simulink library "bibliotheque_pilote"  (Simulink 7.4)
settings: Solver=ode45  StartTime=0.0  StopTime=10.0  RelTol=1e-3
libraries: fl_lib x20, nesl_utility x7, elec_lib x1

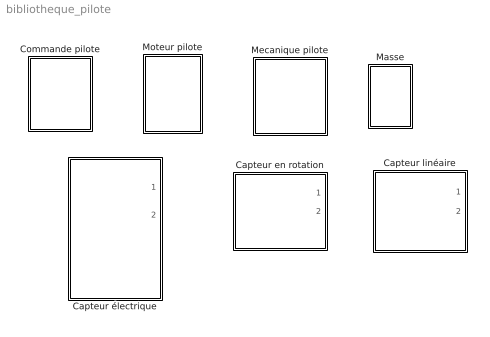
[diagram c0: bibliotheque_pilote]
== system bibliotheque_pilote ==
  Capteur en rotation : Subsystem
  Capteur linéaire : Subsystem
  Capteur électrique : Subsystem
  Commande pilote : Subsystem
  Masse : Subsystem  mask(Masse soulevée par la tige){masse=14}
      mask prompts: masse "Masse en kg"
  Mecanique pilote : Subsystem
  Moteur pilote : Subsystem

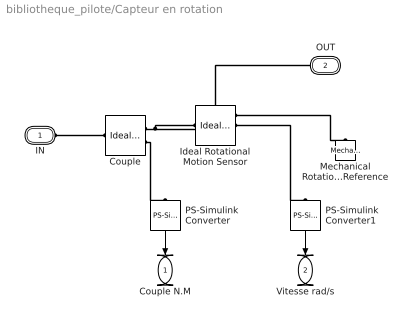
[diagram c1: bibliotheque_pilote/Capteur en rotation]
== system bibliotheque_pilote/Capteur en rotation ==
  Couple : fl_lib/Mechanical/Mechanical Sensors/Ideal Torque Sensor  DialogController=NetworkEngine.DynNeDlgSource  SystemSampleTime=-1  w_Log=off  t_Log=off  LocalVarNames=|w|t  LocalVarDescs=|w|t  LocalVarLogging=[0 0]
  Ideal Rotational Motion Sensor : fl_lib/Mechanical/Mechanical Sensors/Ideal Rotational Motion Sensor  DialogController=NetworkEngine.DynNeDlgSource  SystemSampleTime=-1  offset=0 rad  w_Log=off  t_Log=off  phi_Log=off  LocalVarNames=|w|t|phi  LocalVarDescs=|w|t|phi  LocalVarLogging=[0 0 0]
  Mechanical Rotational Reference : fl_lib/Mechanical/Rotational Elements/Mechanical Rotational Reference  DialogController=NetworkEngine.DynNeDlgSource  SystemSampleTime=-1  t_Log=off  LocalVarNames=|t  LocalVarDescs=|t  LocalVarLogging=0
  PS-Simulink Converter : nesl_utility/PS-Simulink Converter  DialogController=NetworkEngine.DynNeUtilDlgSource  SystemSampleTime=-1  PhysicalDomain=network_engine_domain  LeftPortType=input  RightPortType=output  SubClassName=ps_output  Unit=N*m  AffineConversion=off
  PS-Simulink Converter1 : nesl_utility/PS-Simulink Converter  DialogController=NetworkEngine.DynNeUtilDlgSource  SystemSampleTime=-1  PhysicalDomain=network_engine_domain  LeftPortType=input  RightPortType=output  SubClassName=ps_output  Unit=rad/s  AffineConversion=off
  IN : PMIOPort  Tag=PMCPort  Port=1  Side=Left
  OUT : PMIOPort  Tag=PMCPort  Port=2  Side=Right
  Couple N.M : Outport  OutDataType=fixdt(1, 16)  OutScaling=2^0
  Vitesse rad/s : Outport  Port=2  OutDataType=fixdt(1, 16)  OutScaling=2^0
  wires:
  PS-Simulink Converter/1 -> Couple N.M/1
  PS-Simulink Converter1/1 -> Vitesse rad/s/1
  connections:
  IN/RConn1 -- Couple/LConn1
  Couple/RConn1 -- Ideal Rotational Motion Sensor/LConn1 -- OUT/RConn1
  Couple/RConn2 -- PS-Simulink Converter/LConn1
  Ideal Rotational Motion Sensor/RConn2 -- PS-Simulink Converter1/LConn1
  Ideal Rotational Motion Sensor/RConn1 -- Mechanical Rotational Reference/LConn1

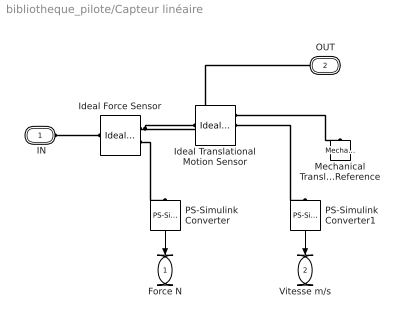
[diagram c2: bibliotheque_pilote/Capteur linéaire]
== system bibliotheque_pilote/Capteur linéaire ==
  Ideal Force Sensor : fl_lib/Mechanical/Mechanical Sensors/Ideal Force Sensor  DialogController=NetworkEngine.DynNeDlgSource  SystemSampleTime=-1  v_Log=off  f_Log=off  LocalVarNames=|v|f  LocalVarDescs=|v|f  LocalVarLogging=[0 0]
  Ideal Translational Motion Sensor : fl_lib/Mechanical/Mechanical Sensors/Ideal Translational Motion Sensor  DialogController=NetworkEngine.DynNeDlgSource  SystemSampleTime=-1  offset=0 m  v_Log=off  f_Log=off  x_Log=off  LocalVarNames=|v|f|x  LocalVarDescs=|v|f|x  LocalVarLogging=[0 0 0]
  Mechanical Translational Reference : fl_lib/Mechanical/Translational Elements/Mechanical Translational Reference  DialogController=NetworkEngine.DynNeDlgSource  SystemSampleTime=-1  f_Log=off  LocalVarNames=|f  LocalVarDescs=|f  LocalVarLogging=0
  PS-Simulink Converter : nesl_utility/PS-Simulink Converter  DialogController=NetworkEngine.DynNeUtilDlgSource  SystemSampleTime=-1  PhysicalDomain=network_engine_domain  LeftPortType=input  RightPortType=output  SubClassName=ps_output  Unit=N  AffineConversion=off
  PS-Simulink Converter1 : nesl_utility/PS-Simulink Converter  DialogController=NetworkEngine.DynNeUtilDlgSource  SystemSampleTime=-1  PhysicalDomain=network_engine_domain  LeftPortType=input  RightPortType=output  SubClassName=ps_output  Unit=m/s  AffineConversion=off
  " IN" : PMIOPort  Tag=PMCPort  Port=1  Side=Left
  OUT : PMIOPort  Tag=PMCPort  Port=2  Side=Right
  Force N : Outport  OutDataType=fixdt(1, 16)  OutScaling=2^0
  Vitesse m/s : Outport  Port=2  OutDataType=fixdt(1, 16)  OutScaling=2^0
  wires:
  PS-Simulink Converter/1 -> Force N/1
  PS-Simulink Converter1/1 -> Vitesse m/s/1
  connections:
  " IN"/RConn1 -- Ideal Force Sensor/LConn1
  Ideal Force Sensor/RConn1 -- Ideal Translational Motion Sensor/LConn1 -- OUT/RConn1
  Ideal Force Sensor/RConn2 -- PS-Simulink Converter/LConn1
  Ideal Translational Motion Sensor/RConn2 -- PS-Simulink Converter1/LConn1
  Ideal Translational Motion Sensor/RConn1 -- Mechanical Translational Reference/LConn1

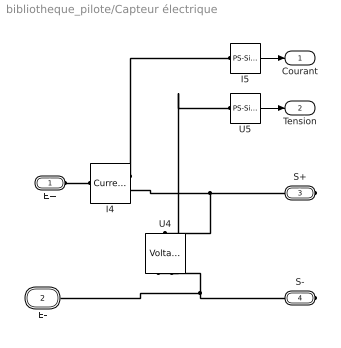
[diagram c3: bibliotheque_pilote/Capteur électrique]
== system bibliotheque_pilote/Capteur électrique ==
  I4 : fl_lib/Electrical/Electrical Sensors/Current Sensor  DialogController=NetworkEngine.DynNeDlgSource  SystemSampleTime=-1  i1_Log=off  v1_Log=off  LocalVarNames=|i1|v1  LocalVarDescs=|i1|v1  LocalVarLogging=[0 0]
  I5 : nesl_utility/PS-Simulink Converter  DialogController=NetworkEngine.DynNeUtilDlgSource  SystemSampleTime=-1  PhysicalDomain=network_engine_domain  LeftPortType=input  RightPortType=output  SubClassName=ps_output  Unit=A  AffineConversion=off
  U4 : fl_lib/Electrical/Electrical Sensors/Voltage Sensor  DialogController=NetworkEngine.DynNeDlgSource  SystemSampleTime=-1  i1_Log=off  v1_Log=off  LocalVarNames=|i1|v1  LocalVarDescs=|i1|v1  LocalVarLogging=[0 0]
  U5 : nesl_utility/PS-Simulink Converter  DialogController=NetworkEngine.DynNeUtilDlgSource  SystemSampleTime=-1  PhysicalDomain=network_engine_domain  LeftPortType=input  RightPortType=output  SubClassName=ps_output  Unit=V  AffineConversion=off
  E+ : PMIOPort  Port=1  Side=Left
  E- : PMIOPort  Port=2  Side=Left
  S+ : PMIOPort  Port=3  Side=Right
  S- : PMIOPort  Port=4  Side=Right
  Courant : Outport
  Tension : Outport  Port=2
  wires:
  U5/1 -> Tension/1
  I5/1 -> Courant/1
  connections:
  S-/RConn1 -- U4/RConn2 -- E-/RConn1
  E+/RConn1 -- I4/LConn1
  U4/RConn1 -- U5/LConn1
  S+/RConn1 -- U4/LConn1 -- I4/RConn2
  I4/RConn1 -- I5/LConn1

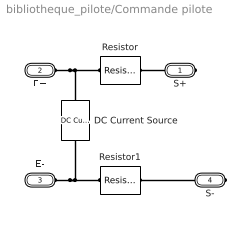
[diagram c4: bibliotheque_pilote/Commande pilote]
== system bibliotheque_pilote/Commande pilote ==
  DC Current Source : fl_lib/Electrical/Electrical Sources/DC Current Source  DialogController=NetworkEngine.DynNeDlgSource  SystemSampleTime=-1  i0=0.2 A  i_Log=off  v_Log=off  LocalVarNames=|i|v  LocalVarDescs=|i|v  LocalVarLogging=[0 0]
  Resistor : fl_lib/Electrical/Electrical Elements/Resistor  DialogController=NetworkEngine.DynNeDlgSource  SystemSampleTime=-1  R=0.7 Ohm  i_Log=off  v_Log=off  LocalVarNames=|i|v  LocalVarDescs=|i|v  LocalVarLogging=[0 0]
  Resistor1 : fl_lib/Electrical/Electrical Elements/Resistor  DialogController=NetworkEngine.DynNeDlgSource  SystemSampleTime=-1  R=1E-6 Ohm  i_Log=off  v_Log=off  LocalVarNames=|i|v  LocalVarDescs=|i|v  LocalVarLogging=[0 0]
  S+ : PMIOPort  Port=1  Side=Right
  E+ : PMIOPort  Port=2  Side=Left
  E- : PMIOPort  Port=3  Side=Left
  S- : PMIOPort  Port=4  Side=Right
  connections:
  E-/RConn1 -- DC Current Source/LConn1 -- Resistor1/RConn1
  E+/RConn1 -- Resistor/LConn1 -- DC Current Source/RConn1
  S+/RConn1 -- Resistor/RConn1
  S-/RConn1 -- Resistor1/LConn1

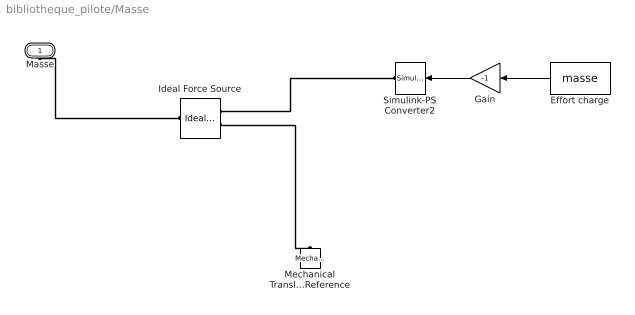
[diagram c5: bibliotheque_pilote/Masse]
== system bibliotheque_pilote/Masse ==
  Effort charge : Constant  Value=masse
  Gain : Gain  Gain=-1  ParameterDataType=fixdt(1, 16)  ParameterScaling=2^0  OutDataType=fixdt(1, 16)  OutScaling=2^0
  Ideal Force Source : fl_lib/Mechanical/Mechanical Sources/Ideal Force Source  DialogController=NetworkEngine.DynNeDlgSource  SystemSampleTime=-1  v_Log=off  f_Log=off  LocalVarNames=|v|f  LocalVarDescs=|v|f  LocalVarLogging=[0 0]
  Mechanical Translational Reference : fl_lib/Mechanical/Translational Elements/Mechanical Translational Reference  DialogController=NetworkEngine.DynNeDlgSource  SystemSampleTime=-1  f_Log=off  LocalVarNames=|f  LocalVarDescs=|f  LocalVarLogging=0
  Simulink-PS Converter2 : nesl_utility/Simulink-PS Converter  DialogController=NetworkEngine.DynNeUtilDlgSource  SystemSampleTime=-1  PhysicalDomain=network_engine_domain  LeftPortType=input  RightPortType=output  SubClassName=ps_input  Unit=N  AffineConversion=off  InputFilterTimeConstant=.001  UdotUserProvided=0
  Masse : PMIOPort  Port=1  Side=Left
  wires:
  Effort charge/1 -> Gain/1
  Gain/1 -> Simulink-PS Converter2/1
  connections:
  Ideal Force Source/RConn2 -- Mechanical Translational Reference/LConn1
  Ideal Force Source/RConn1 -- Simulink-PS Converter2/RConn1
  Ideal Force Source/LConn1 -- Masse/RConn1

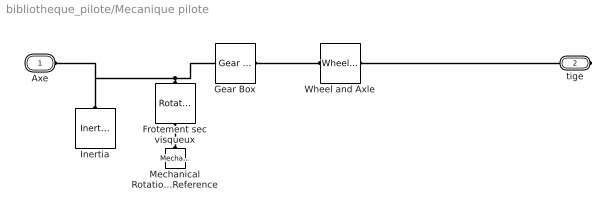
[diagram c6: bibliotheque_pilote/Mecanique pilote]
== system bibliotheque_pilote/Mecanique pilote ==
  Frotement sec visqueux : fl_lib/Mechanical/Rotational Elements/Rotational Friction  DialogController=NetworkEngine.DynNeDlgSource  SystemSampleTime=-1  brkwy_trq=0.01337 N*m  Col_trq=0.01337 N*m  visc_coef=20e-6 N*m/(rad/s)  trans_coef=10 s/rad  vel_thr=1e-5 rad/s  t_Log=off  w_Log=off  LocalVarNames=|t|w  LocalVarDescs=|t|w  LocalVarLogging=[0 0]
  Gear Box : fl_lib/Mechanical/Mechanisms/Gear Box  DialogController=NetworkEngine.DynNeDlgSource  SystemSampleTime=-1  ratio=20/71  t_in_Log=off  t_out_Log=off  LocalVarNames=|t_in|t_out  LocalVarDescs=|t_in|t_out  LocalVarLogging=[0 0]
  Inertia : fl_lib/Mechanical/Rotational Elements/Inertia  DialogController=NetworkEngine.DynNeDlgSource  SystemSampleTime=-1  inertia=2.68e-6 kg*m^2  initial_velocity=0 rad/s  t_Log=off  LocalVarNames=|t  LocalVarDescs=|t  LocalVarLogging=0
  Mechanical Rotational Reference : fl_lib/Mechanical/Rotational Elements/Mechanical Rotational Reference  DialogController=NetworkEngine.DynNeDlgSource  SystemSampleTime=-1  t_Log=off  LocalVarNames=|t  LocalVarDescs=|t  LocalVarLogging=0
  Wheel and Axle : fl_lib/Mechanical/Mechanisms/Wheel and Axle  DialogController=NetworkEngine.DynNeDlgSource  SystemSampleTime=-1  R=0.003/2/3.14 m  or=1  torque_A_Log=off  force_P_Log=off  ang_velocity_Log=off  velocity_Log=off  LocalVarNames=|torque_A|force_P|ang_velocity|velocity  LocalVarDescs=|Axle torque (N*m)|Periphery force (N)|Axle angular velocity (rad/s)|Periphery velocity (m/s)  LocalVarLogging=[0 0 0 0]
  Axe : PMIOPort  Tag=PMCPort  Port=1  Side=Left
  tige : PMIOPort  Port=2  Side=Right
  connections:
  Inertia/LConn1 -- Axe/RConn1 -- Gear Box/LConn1 -- Frotement sec visqueux/LConn1
  Gear Box/RConn1 -- Wheel and Axle/LConn1
  Wheel and Axle/RConn1 -- tige/RConn1
  Mechanical Rotational Reference/LConn1 -- Frotement sec visqueux/RConn1

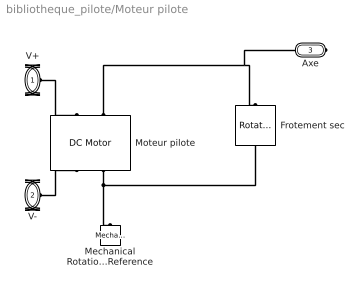
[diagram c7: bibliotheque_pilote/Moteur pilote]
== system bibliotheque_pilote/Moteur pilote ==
  Frotement sec : fl_lib/Mechanical/Rotational Elements/Rotational Friction  DialogController=NetworkEngine.DynNeDlgSource  SystemSampleTime=-1  brkwy_trq=5.43e-3 N*m  Col_trq=5.43e-3 N*m  visc_coef=0 N*m/(rad/s)  trans_coef=10 s/rad  vel_thr=1e-04 rad/s  t_Log=off  w_Log=off  LocalVarNames=|t|w  LocalVarDescs=|t|w  LocalVarLogging=[0 0]
  Mechanical Rotational Reference : fl_lib/Mechanical/Rotational Elements/Mechanical Rotational Reference  DialogController=NetworkEngine.DynNeDlgSource  SystemSampleTime=-1  t_Log=off  LocalVarNames=|t  LocalVarDescs=|t  LocalVarLogging=0
  Moteur pilote : elec_lib/Actuators & Drivers/DC Motor  DialogController=NetworkEngine.DynNeDlgSource  SystemSampleTime=-1  parameterization=1  Ra=1 Ohm  La=1.987e-03 H  emf_or_torque=1  Kv=0.0221 V/(rad/s)  Ki=6.876e-04 N*m/A  T_stall=2.4e-04 N*m  w_max=1.91e+04 rpm  w_rated=1.5e+04 rpm  P_rated=0.08 W  V_rated=1.5 V  J=9.32e-6 kg*m^2  lam=0.397e-07 N*m/(rad/s)  speed0=0 rpm  current_Log=off  voltage_Log=off  power_Log=off  i2r_Log=off  torque_Log=off  speed_Log=off  LocalVarNames=|current|voltage|power|i2r|torque|speed  LocalVarDescs=|Current (A)|Voltage (V)|Power (W)|Electrical losses (W)|Torque (Nm)|Angular speed (rad/s)  LocalVarLogging=[0 0 0 0 0 0]
  V+ : PMIOPort  Port=1  Side=Left
  V- : PMIOPort  Port=2  Side=Left
  Axe : PMIOPort  Port=3  Side=Right
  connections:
  Moteur pilote/RConn2 -- Mechanical Rotational Reference/LConn1 -- Frotement sec/RConn1
  V+/RConn1 -- Moteur pilote/LConn1
  V-/RConn1 -- Moteur pilote/RConn1
  Moteur pilote/LConn2 -- Axe/RConn1 -- Frotement sec/LConn1
